FUNCTION FC 110 : VOID
TITLE =
VERSION : 0.1

BEGIN
NETWORK
TITLE =Abilita/reset richiesta accesso scarto cc1
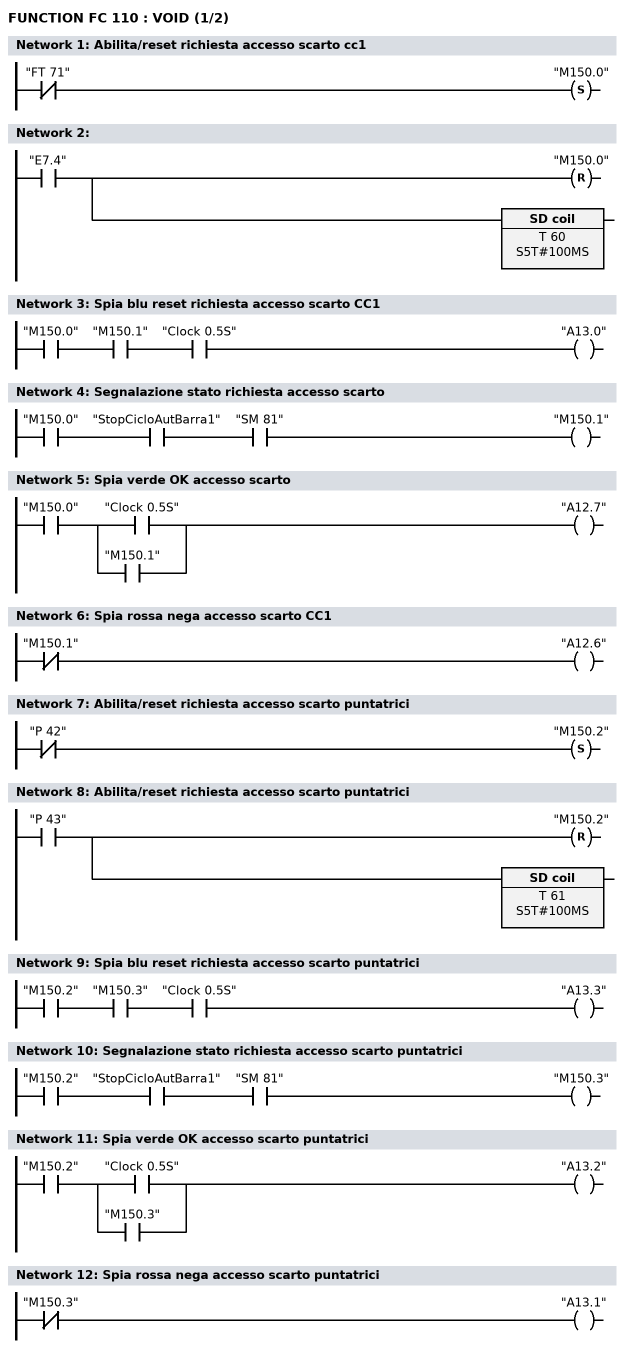
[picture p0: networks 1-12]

      UN    "FT 71";
      S     "M150.0";
NETWORK
TITLE =

      U     "E7.4";
      R     "M150.0";
      L     S5T#100MS;
      SE    T     60;
NETWORK
TITLE =Spia blu reset richiesta accesso scarto CC1

      U     "M150.0";
      U     "M150.1";
      U     "Clock 0.5S";
      =     "A13.0";
NETWORK
TITLE =Segnalazione stato richiesta accesso scarto

      U     "M150.0";
      U     "StopCicloAutBarra1";
      U     "SM 81";
      =     "M150.1";
NETWORK
TITLE =Spia verde OK accesso scarto

      U     "M150.0";
      U(    ;
      O     "Clock 0.5S";
      O     "M150.1";
      )     ;
      =     "A12.7";
NETWORK
TITLE =Spia rossa nega accesso scarto CC1

      UN    "M150.1";
      =     "A12.6";
NETWORK
TITLE =Abilita/reset richiesta accesso scarto puntatrici

      UN    "P 42";
      S     "M150.2";
NETWORK
TITLE =Abilita/reset richiesta accesso scarto puntatrici

      U     "P 43";
      R     "M150.2";
      L     S5T#100MS;
      SE    T     61;
NETWORK
TITLE =Spia blu reset richiesta accesso scarto puntatrici

      U     "M150.2";
      U     "M150.3";
      U     "Clock 0.5S";
      =     "A13.3";
NETWORK
TITLE =Segnalazione stato richiesta accesso scarto puntatrici

      U     "M150.2";
      U     "StopCicloAutBarra1";
      U     "SM 81";
      =     "M150.3";
NETWORK
TITLE =Spia verde OK accesso scarto puntatrici

      U     "M150.2";
      U(    ;
      O     "Clock 0.5S";
      O     "M150.3";
      )     ;
      =     "A13.2";
NETWORK
TITLE =Spia rossa nega accesso scarto puntatrici

      UN    "M150.3";
      =     "A13.1";
NETWORK
TITLE =Abilita/reset richiesta accesso scarto prova tenuta
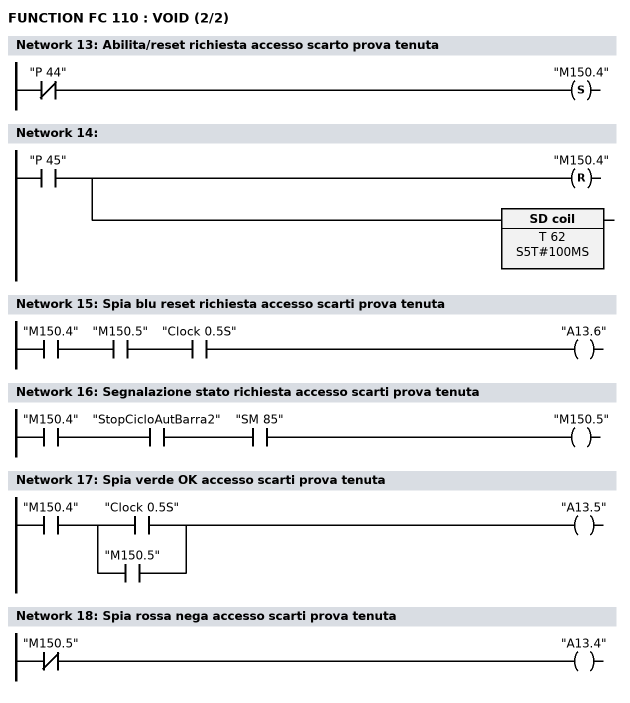
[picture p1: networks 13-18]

      UN    "P 44";
      S     "M150.4";
NETWORK
TITLE =

      U     "P 45";
      R     "M150.4";
      L     S5T#100MS;
      SE    T     62;
NETWORK
TITLE =Spia blu reset richiesta accesso scarti prova tenuta

      U     "M150.4";
      U     "M150.5";
      U     "Clock 0.5S";
      =     "A13.6";
NETWORK
TITLE =Segnalazione stato richiesta accesso scarti prova tenuta

      U     "M150.4";
      U     "StopCicloAutBarra2";
      U     "SM 85";
      =     "M150.5";
NETWORK
TITLE =Spia verde OK accesso scarti prova tenuta

      U     "M150.4";
      U(    ;
      O     "Clock 0.5S";
      O     "M150.5";
      )     ;
      =     "A13.5";
NETWORK
TITLE =Spia rossa nega accesso scarti prova tenuta

      UN    "M150.5";
      =     "A13.4";
END_FUNCTION

